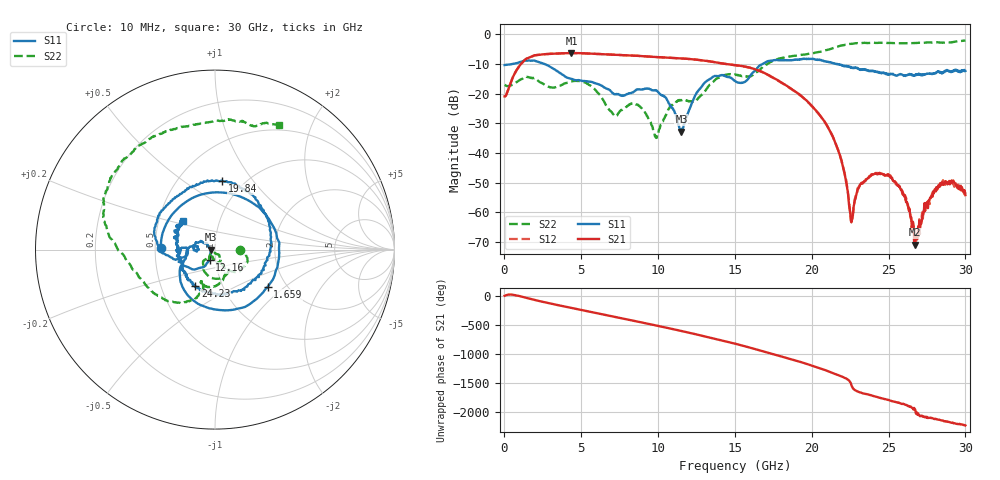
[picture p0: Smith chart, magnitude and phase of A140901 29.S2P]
!  2-Port S-parameters saved by WinCal
! VAR MeasName=S-Parameters (CALIBRATED_DATA) read from VNA (N5244A)
! VAR MeasDate=11/3/2014 9:29:10 AM
! VAR NAME=A140901 29
! VAR FILENAME=A140901 29.S2P
! VAR DATE=11/3/2014 9:29:10 AM
! VAR PHYS_PORTS=1,2
# Hz S RI R 50
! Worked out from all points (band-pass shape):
!   801 points, 10 MHz to 30 GHz, reference 50 ohm
!   highest |S21| = -6.34 dB at 4.359 GHz (marker M1); lowest = -70.9 dB at 26.7 GHz (marker M2)
!   |S21| within 3 dB of the highest: 1.195 GHz to 13.59 GHz (12.4 GHz wide, 168 % of centre)
!   lowest |S11| = -32.8 dB at 11.52 GHz (marker M3), VSWR 1.05, Z = 47.8 - j0.0614 ohm
!   |S11| at or under -10 dB: start of sweep to 526.1 MHz; 2.592 GHz to 16.82 GHz (14.23 GHz wide, 147 % of centre); 21.65 GHz to end of sweep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
!   |S22| runs from -34.9 to -2.1 dB; largest |S21 - S12| = 0.0034
!   S11 on the Smith chart (normalised r, x): 10 MHz: 0.54, +0.01; 1.659 GHz: 1.61, -0.76; 12.16 GHz: 0.94, -0.11; 19.84 GHz: 0.80, +0.72; 24.23 GHz: 0.74, -0.32; 30 GHz: 0.67, +0.23
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1e7  -0.3028 0.00767  0.0897 0.00225  0.0895 0.00213  0.1409 -0.00136
7.5975e8  0.0946 0.31  0.2384 0.0393  0.2382 0.0397  0.1547 -0.00581
1.65945e9  0.2938 -0.2068  0.2655 -0.3134  0.2658 -0.3135  0.1593 -0.0972
4.35855e9  -0.1684 -0.0559  -0.4286 0.2202  -0.4287 0.2212  0.0496 -0.152
5.033325e9  -0.1612 -0.0333  -0.2067 0.4315  -0.206 0.4313  -0.014 -0.1592
7.245088e9  -0.0959 0.0172  0.45 -0.0289  0.4494 -0.0282  -0.0141 -0.0387
8.669612e9  -0.1175 -0.00261  0.0644 -0.4282  0.0642 -0.4279  -0.0318 -0.0558
1.001916e10  -0.0983 0.0393  -0.3766 -0.1665  -0.3761 -0.1659  0.00356 -0.0216
1.151866e10  -0.0229 -0.000642  -0.182 0.3459  -0.1815 0.3452  0.0222 -0.074
1.215595e10  -0.0297 -0.0574  0.0691 0.3741  0.0683 0.3736  0.0174 -0.0718
1.346801e10  -0.1563 -0.0957  0.3449 -0.00959  0.3444 -0.0103  0.0585 -0.1358
1.5005e10  -0.1626 0.0116  -0.0494 -0.2973  -0.0506 -0.2956  -0.0637 -0.1988
1.702932e10  -0.3321 0.0702  -0.0856 0.1967  -0.0851 0.1951  -0.1238 -0.2822
1.984089e10  0.0417 0.3806  -0.0136 -0.0676  -0.0127 -0.067  -0.4575 -0.11
2.002832e10  0.0901 0.3754  -0.0278 -0.0543  -0.0271 -0.0545  -0.4671 -0.0936
2.167778e10  0.3094 0.0299  0.000779 0.0118  0.000675 0.0118  -0.6035 0.1202
2.257748e10  0.2119 -0.1684  6.16e-08 -0.000684  0.000121 -0.000671  -0.6083 0.3255
2.422692e10  -0.1099 -0.2033  0.00164 0.00407  0.00186 0.0041  -0.3829 0.6038
2.501416e10  -0.1673 -0.1233  0.00423 0.000962  0.00417 0.000825  -0.2618 0.6643
2.67011e10  -0.199 -0.0161  -0.000221 -0.00018  -0.000497 -0.000156  -0.0412 0.7082
2.838804e10  -0.2179 0.0738  0.00252 0.00133  0.00248 0.00141  0.1875 0.6996
3e10  -0.1792 0.1603  0.000895 -0.00173  0.00113 -0.00188  0.3586 0.6969
